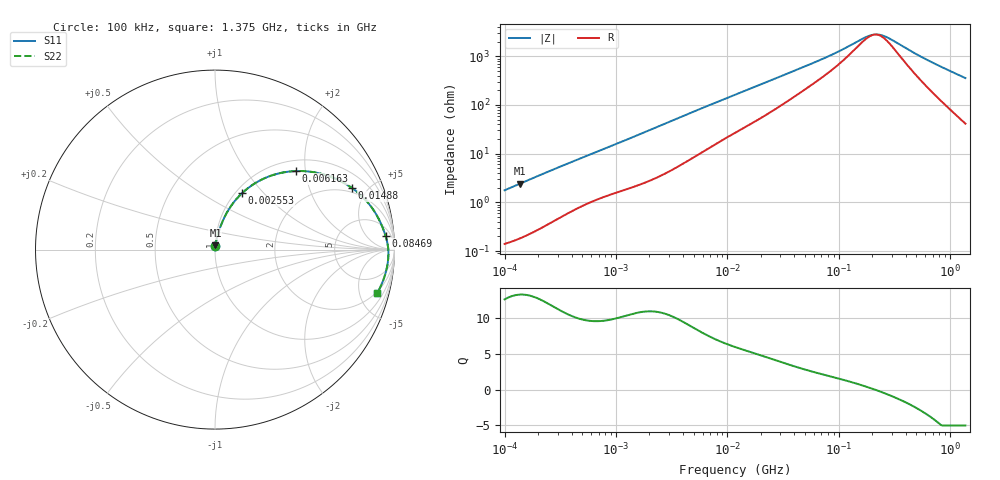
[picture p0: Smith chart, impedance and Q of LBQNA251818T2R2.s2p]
! LBQNA251818T2R2  S-PARAMETER MODEL  ( General Type )
! Model Generated by TAIYO YUDEN Corporation (http://www.ty-top.com)
! Version 1.0
! TAIYO YUDEN Control No. 191025NI43SB-FBB
! Copyright(c) 2019 TAIYO YUDEN CO.,LTD. All Rights Reserved.
! Product Description (link to TY-COMPAS)
! https://ds.yuden.co.jp/TYCOMPAS/or/detail?pn=LBQNA251818T2R2M&u=M
! Products Name : Inductors
! Characteristics :
!  Inductance : 2.2 uH , SRF(min) : 68 MHz , DC Resistance(max) : 0.117 Ohm
!  Rated Current : Saturation :510 mA , Temp Rise : 1000 mA (20 degC)
!  Case Size : 2.5 x 1.8 / 0.098 x 0.071 [mm/inch] , Thickness : 1.8 / 0.071 [mm/inch]
!  (Conditions: Temperature = 25 degC , DC Bias Current/Voltage = 0A / 0V)
! External Node Assignments :
!  1  o---GGG---o  2
! GND o---------o GND
! Frequency Range : 0.1MHz  -  1374.841115MHz  [ 402 STEP ]
# MHz S RI R 50
! Freq[MHz].  S11 Real  S11 Imag  S21 Real  S21 Imag  S12 Real  S12 Imag  S22 Real  S22 Imag
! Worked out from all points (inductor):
!   401 points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, 100 kHz to 1.375 GHz, reference 50 ohm
!   read as one part in series: L = 2.8 uH near 104.9 kHz
!   highest Q = 13.3 at 136.3 kHz (marker M1), where L = 2.8 uH
!   self-resonance near 212.1 MHz
!   S11 on the Smith chart (normalised r, x): 100 kHz: 1.00, +0.04; 2.553 MHz: 1.07, +0.76; 6.163 MHz: 1.23, +1.77; 14.88 MHz: 1.73, +3.95; 84.69 MHz: 11, +18; 1.375 GHz: 1.83, -7.10
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0.1  0.00171 0.0176  0.9983 -0.0176  0.9983 -0.0176  0.00171 0.0176
0.136299  0.00237 0.0238  0.9976 -0.0238  0.9976 -0.0238  0.00237 0.0238
0.493352  0.0147 0.0797  0.9853 -0.0797  0.9853 -0.0797  0.0147 0.0797
1.27933  0.054 0.183  0.946 -0.183  0.946 -0.183  0.054 0.183
2.433966  0.14 0.3039  0.86 -0.3039  0.86 -0.3039  0.14 0.3039
2.552736  0.1502 0.3138  0.8498 -0.3138  0.8498 -0.3138  0.1502 0.3138
3.827204  0.2644 0.3922  0.7356 -0.3922  0.7356 -0.3922  0.2644 0.3922
6.163029  0.4493 0.4377  0.5507 -0.4377  0.5507 -0.4377  0.4493 0.4377
8.400157  0.5749 0.4265  0.4251 -0.4265  0.4251 -0.4265  0.5749 0.4265
11.72536  0.6941 0.3845  0.3059 -0.3845  0.3059 -0.3845  0.6941 0.3845
14.8793  0.7636 0.3428  0.2364 -0.3428  0.2364 -0.3428  0.7636 0.3428
26.99127  0.8773 0.2287  0.1227 -0.2287  0.1227 -0.2287  0.8773 0.2287
57.84736  0.9367 0.1158  0.0633 -0.1158  0.0633 -0.1158  0.9367 0.1158
84.6864  0.9503 0.0763  0.0497 -0.0763  0.0497 -0.0763  0.9503 0.0763
165.0028  0.9634 0.0199  0.0366 -0.0199  0.0366 -0.0199  0.9634 0.0199
194.9444  0.965 0.0067  0.035 -0.0067  0.035 -0.0067  0.965 0.0067
214.4338  0.9656 -0.000888  0.0344 0.000888  0.0344 0.000888  0.9656 -0.000888
235.8717  0.966 -0.00856  0.034 0.00856  0.034 0.00856  0.966 -0.00856
285.3914  0.9662 -0.0244  0.0338 0.0244  0.0338 0.0244  0.9662 -0.0244
611.6473  0.9572 -0.1031  0.0428 0.1031  0.0428 0.1031  0.9572 -0.1031
961.7629  0.937 -0.1719  0.063 0.1719  0.063 0.1719  0.937 -0.1719
1374.841  0.9031 -0.2432  0.0969 0.2432  0.0969 0.2432  0.9031 -0.2432
